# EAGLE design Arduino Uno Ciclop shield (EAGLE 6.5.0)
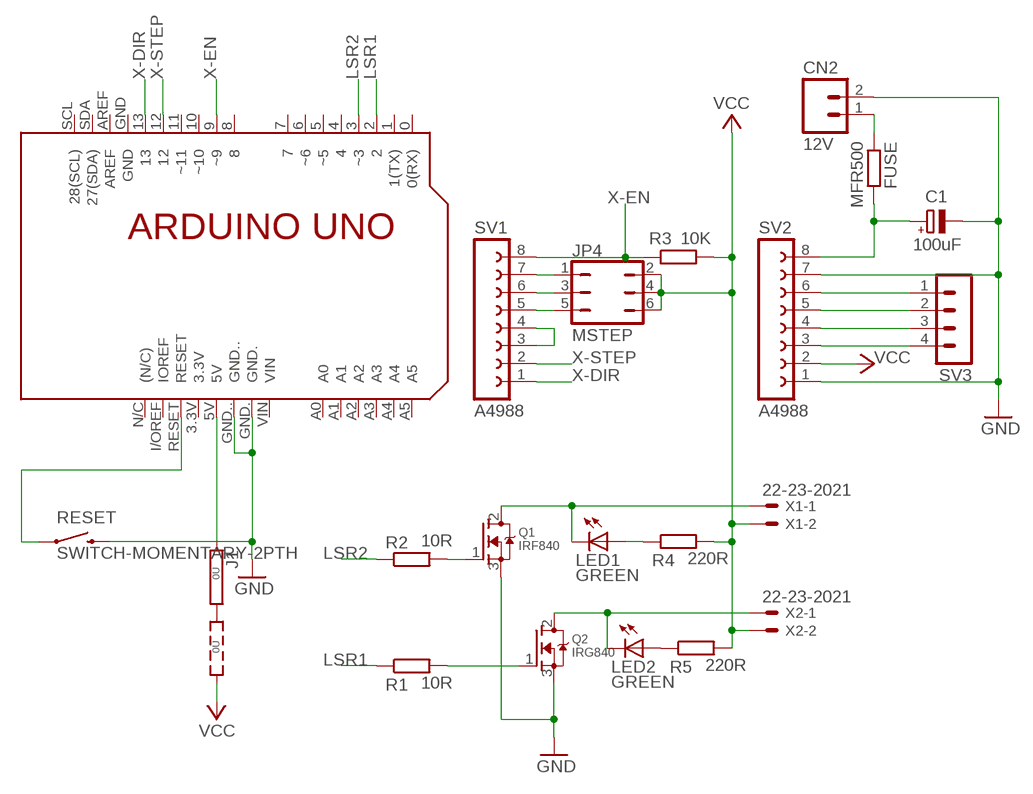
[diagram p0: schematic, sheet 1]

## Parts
C1  100uF  CPOL-EUB45181A  [B45181A]
CN2  12V  M025MM  [SCREWTERMINAL-5MM-2]
FUSE  MFR500  R-EU_0207/10  [0207/10]
J1  0R2  [0R2/10]
JP4  MSTEP  JP3Q  [JP3Q]
LED1  GREEN  LED5MM  [LED5MM]
LED2  GREEN  LED5MM  [LED5MM]
PCB1  ARDUINO_UNO  [ARDUINO_UNO]
Q1  IRF840  MOSFET-NGDS_TO220V  [TO220V]
Q2  IRG840  MOSFET-NGDS_TO220V  [TO220V]
R1  10R  R-EU_0207/10  [0207/10]
R2  10R  R-EU_0207/10  [0207/10]
R3  10K  R-EU_0207/10  [0207/10]
R4  220R  R-EU_0207/10  [0207/10]
R5  220R  R-EU_0207/10  [0207/10]
RESET  SWITCH-MOMENTARY-2PTH  [TACTILE-PTH]
SV1  A4988  FE08-1  [FE08]
SV2  A4988  FE08-1  [FE08]
SV3  MA04-1  [MA04-1]
X1  22-23-2021  [22-23-2021]
X2  22-23-2021  [22-23-2021]

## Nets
GND: C1.- CN2.2 PCB1.GND. PCB1.GND.. Q1.3(S) Q2.3(S) RESET.3 SV2.1 SV2.7
LSR1: PCB1.2 R1.1
LSR2: PCB1.3(~3) R2.1
N$1: LED2.A R5.1
N$2: SV2.6 SV3.1
N$3: SV2.5 SV3.2
N$4: SV2.4 SV3.3
N$5: SV2.3 SV3.4
N$6: Q1.1(G) R2.2
N$7: PCB1.RESET RESET.1
N$8: JP4.1 SV1.7
N$9: LED1.K(C) Q1.2(D) X1.1
N$10: JP4.3 SV1.6
N$11: JP4.5 SV1.5
N$12: C1.+ FUSE.2 SV2.8
N$13: CN2.1 FUSE.1
N$14: Q2.1(G) R1.2
N$15: SV1.3 SV1.4
N$16: LED2.K(C) Q2.2(D) X2.1
N$17: LED1.A R4.1
N$18: J1.1 PCB1.5V
VCC: J1.3 JP4.2 JP4.4 JP4.6 R3.2 R4.2 R5.2 SV2.2 X1.2 X2.2
X-DIR: PCB1.13 SV1.1
X-EN: PCB1.9(~9) R3.1 SV1.8
X-STEP: PCB1.12 SV1.2
Unconnected: J1.2 PCB1.0(0(RX)) PCB1.1(1(TX)) PCB1.3.3V PCB1.4 PCB1.5(~5) PCB1.6(~6) PCB1.7 PCB1.8 PCB1.10(~10) PCB1.11(~11) PCB1.A0 PCB1.A1 PCB1.A2 PCB1.A3 PCB1.A4 PCB1.A5 PCB1.AREF PCB1.GND PCB1.I/OREF(IOREF) PCB1.N/C((N/C)) PCB1.SCL(28(SCL)) PCB1.SDA(27(SDA)) PCB1.VIN

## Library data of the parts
C1 = rcl:CPOL-EU: POLARIZED CAPACITOR, European symbol
CN2 = SparkFun-Connectors:M02: Standard 2-pin 0.1" header. Use with; STOREFRONT_ID: PRT-08432
FUSE R1-R5 = resistor:R-EU_: RESISTOR, European symbol
J1 = jumper:0R2: Bridge switch 0R 2 x 10mm
JP4 = jumper:JP3Q: JUMPER
LED1 LED2 = led:LED: LED
PCB1 = E14_Arduino_revB:ARDUINO_UNO: Device for representing an Arduino Uno board with a footprint in an EAGLE design. Created by Dave Young for Element14. More EAGLE documentation at: http://www.element14.com/community/community/knode/cadsoft_eagle
Q1 Q2 = adafruit:MOSFET-N: N-Channel Mosfet 2N7002E - 60V 260mA SOT23 [Digikey: 2N7002ET1GOSTR-ND] - REEL BSH103 - 30V 850mA SOT23 [Digikey: 568-5013-1-ND]
RESET = SparkFun-Electromechanical:SWITCH-MOMENTARY-2: Various NO switches- pushbuttons, reed, etc; PROD_ID: SWCH-08441
SV1 SV2 = con-lsta:FE08-1: FEMALE HEADER; OC_FARNELL: unknown; OC_NEWARK: unknown
SV3 = con-lstb:MA04-1: PIN HEADER; OC_FARNELL: unknown; OC_NEWARK: unknown
X1 X2 = con-molex:22-23-2021: .100" (2.54mm) Center Header - 2 Pin; MF: MOLEX; MPN: 22-23-2021; OC_FARNELL: 1462926; OC_NEWARK: 25C3832

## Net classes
0 default: width 0.024 mm

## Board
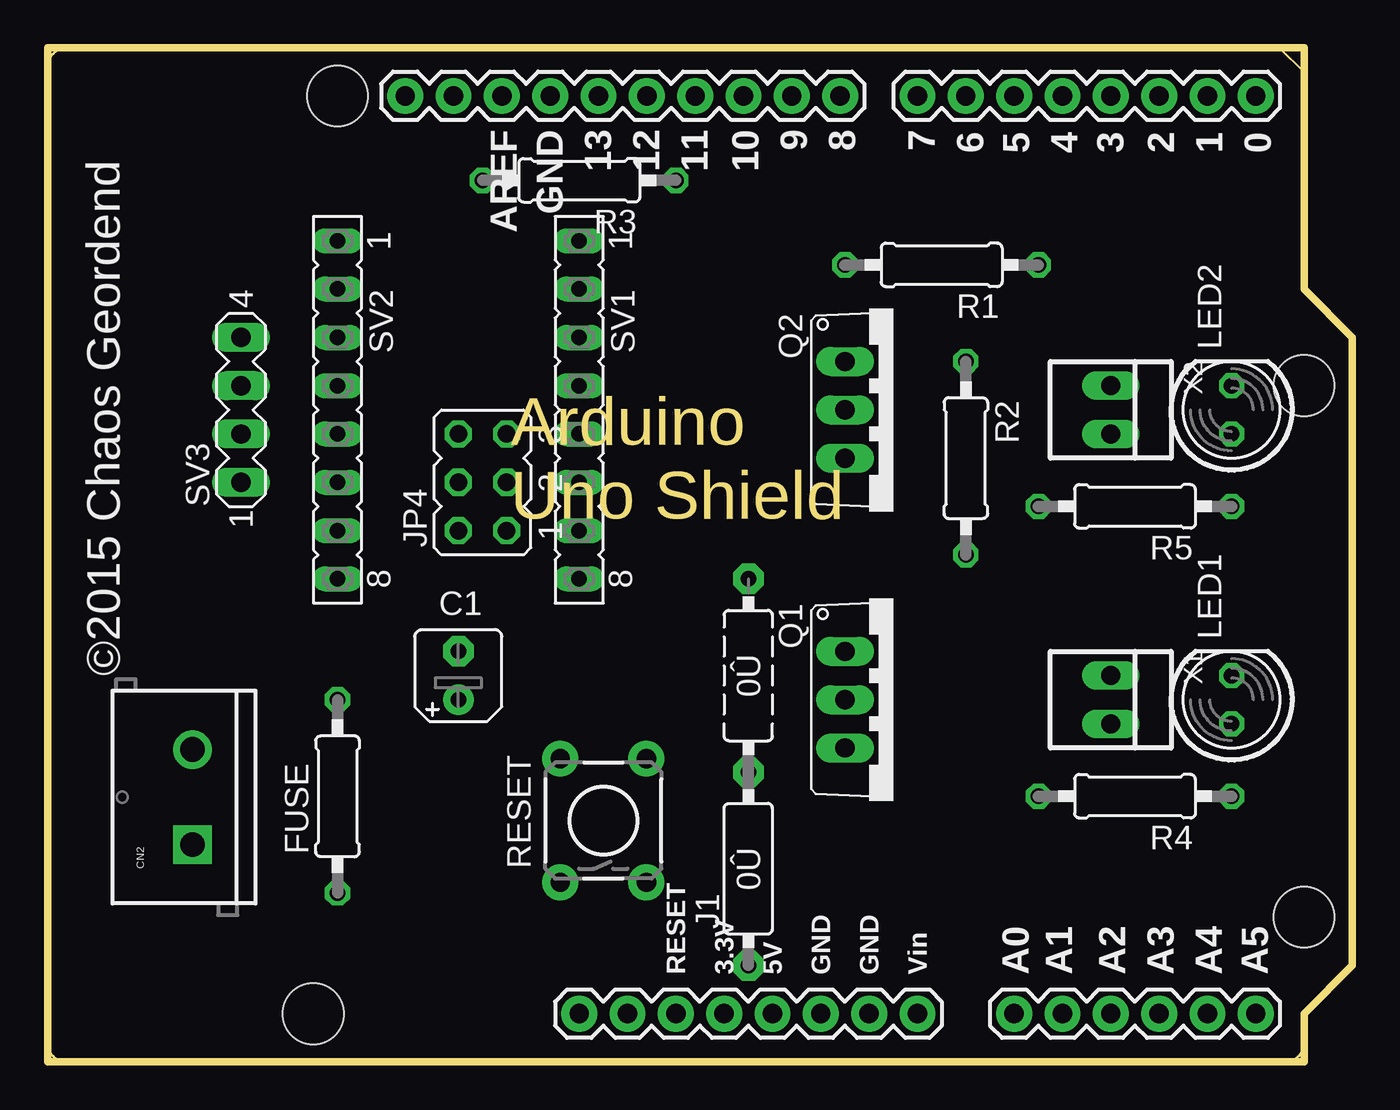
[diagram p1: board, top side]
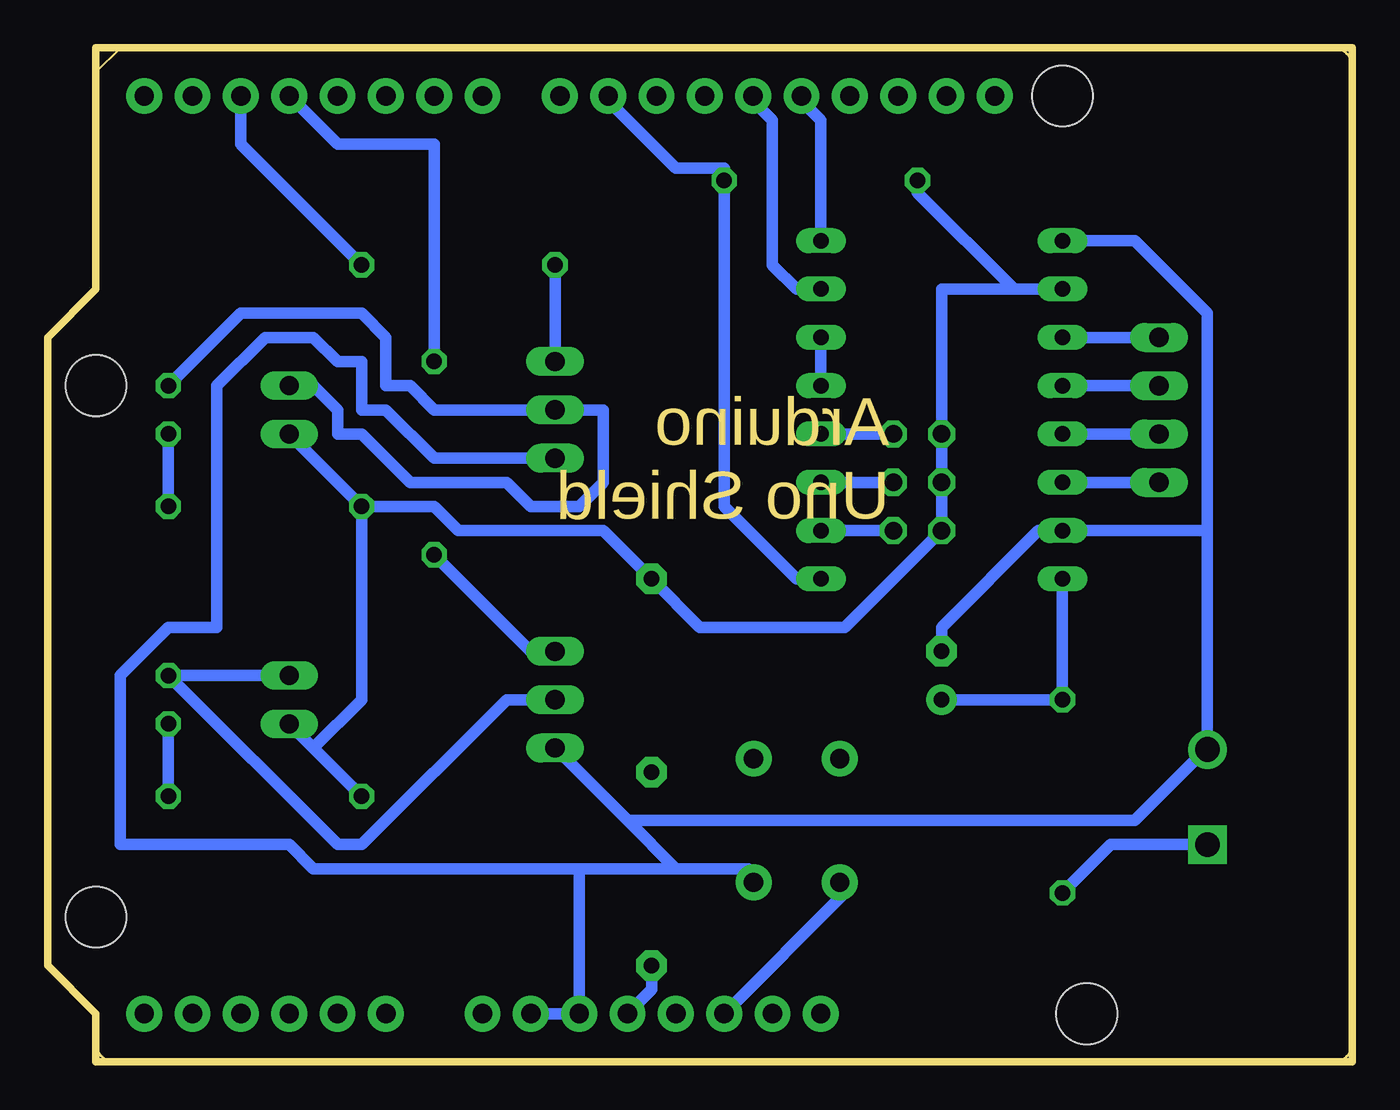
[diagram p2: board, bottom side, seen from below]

Size 68.58 x 53.34 mm. Coordinates in mm from the lower left corner, seen from the top.
Outline: 0,0 0,53.34 66.04,53.34 66.04,40.64 68.58,38.1 68.58,5.08 66.04,2.54 66.04,0 0,0
Copper layers (1*16): Top 0.035mm / dielectric 1.5mm / Bottom 0.035mm
Design rules "default *": minimum track width 24mil, minimum drill 24mil, track to track 16mil, track to pad 16mil, pad to pad 8mil, via to via 8mil, smd to smd 8mil, copper to edge 40mil, drill to drill 8mil, minimum pad ring 10mil, minimum via ring 8mil, stop-mask expansion 4mil, vias tented up to drill 0mil, thermal gap 10mil

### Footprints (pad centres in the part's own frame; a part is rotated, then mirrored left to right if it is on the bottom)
B45181A = drill 0.813 pad 1.6: + -1.27,0 | drill 0.813 pad 1.6 octagon: - 1.27,0
SCREWTERMINAL-5MM-2 = drill 1.3 pad 2.032 square: 1 0,0 | drill 1.3 pad 2.032: 2 5,0
0207/10 = drill 0.813 octagon: 1 -5.08,0; 2 5.08,0
0R2/10 = drill 0.813 pad 1.6 octagon: 1 -5.08,0; 2 5.08,0; 3 15.24,0
JP3Q = drill 0.914 octagon: 1 -2.54,-1.27; 2 -2.54,1.27; 3 0,-1.27; 4 0,1.27; 5 2.54,-1.27; 6 2.54,1.27
LED5MM = drill 0.813 octagon: A -1.27,0; K 1.27,0
ARDUINO_UNO = drill 1.016 pad 1.88: 0 63.5,50.8; 1 60.96,50.8; 2 58.42,50.8; 3 55.88,50.8; 3.3V 35.56,2.54; 4 53.34,50.8; 5 50.8,50.8; 5V 38.1,2.54; 6 48.26,50.8; 7 45.72,50.8; 8 41.656,50.8; 9 39.116,50.8; 10 36.576,50.8; 11 34.036,50.8; 12 31.496,50.8; 13 28.956,50.8; A0 50.8,2.54; A1 53.34,2.54; A2 55.88,2.54; A3 58.42,2.54; A4 60.96,2.54; A5 63.5,2.54; AREF 23.876,50.8; GND 26.416,50.8; GND. 43.18,2.54; GND.. 40.64,2.54; I/OREF 30.48,2.54; N/C 27.94,2.54; RESET 33.02,2.54; SCL 18.796,50.8; SDA 21.336,50.8; VIN 45.72,2.54 | hole 3.2: 66.04,7.62; 66.04,35.56; 15.24,50.8; 13.97,2.54
TO220V = drill 1.016 long: 1 -2.54,-2.54; 2 0,-2.54; 3 2.54,-2.54
TACTILE-PTH = drill 1.016 pad 1.88: 1 -3.251,2.261; 2 3.251,2.261; 3 -3.251,-2.261; 4 3.251,-2.261
FE08 = drill 0.813 long: 1 -8.89,0; 2 -6.35,0; 3 -3.81,0; 4 -1.27,0; 5 1.27,0; 6 3.81,0; 7 6.35,0; 8 8.89,0
MA04-1 = drill 1.016 long: 1 -3.81,0; 2 -1.27,0; 3 1.27,0; 4 3.81,0
22-23-2021 = drill 1 long: 1 -1.27,0; 2 1.27,0

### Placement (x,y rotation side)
C1  21.59,20.32 90 top
CN2  7.62,11.43 90 top
FUSE  15.24,13.97 90 top
J1  36.83,10.16 90 top
JP4  22.86,30.48 90 top
LED1  62.23,19.05 90 top
LED2  62.23,34.29 90 top
PCB1  0,0 0 top
Q1  44.45,19.05 270 top
Q2  44.45,34.29 270 top
R1  46.99,41.91 180 top
R2  48.26,31.75 270 top
R3  27.94,46.35 180 top
R4  57.15,13.97 180 top
R5  57.15,29.21 180 top
RESET  29.21,12.7 90 top
SV1  27.94,34.29 270 top
SV2  15.24,34.29 270 top
SV3  10.16,34.29 90 top
X1  55.88,19.05 270 top
X2  55.88,34.29 270 top

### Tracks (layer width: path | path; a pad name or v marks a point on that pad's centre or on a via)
GND
  Bottom 0.61: C1.- 21.59,22.86 16.51,27.94 SV2.7 7.62,27.94 | SV2.1 11.43,43.18 7.62,39.37 7.62,27.94 | 7.62,27.94 7.62,16.51 | PCB1.GND. PCB1.GND.. 40.64,10.16 | 35.56,10.16 38.1,12.7 | 38.1,12.7 Q1.3 | 35.56,10.16 31.75,10.16 RESET.3 | Q2.3 48.26,31.75 50.8,34.29 52.07,34.29 52.07,36.83 53.34,36.83 54.61,38.1 57.15,38.1 59.69,35.56 59.69,22.86 62.23,22.86 64.77,20.32 64.77,11.43 55.88,11.43 54.61,10.16 40.64,10.16 | 35.56,10.16 40.64,10.16 | 7.62,16.51 11.43,12.7 38.1,12.7 | 7.62,16.51 CN2.2
LSR1
  Bottom 0.61: R1.1 58.42,48.26 PCB1.2
LSR2
  Bottom 0.61: R2.1 48.26,48.26 53.34,48.26 PCB1.3
N$1
  Bottom 0.61: LED2.A R5.1
N$2
  Bottom 0.61: SV3.1 SV2.6
N$3
  Bottom 0.61: SV3.2 SV2.5
N$4
  Bottom 0.61: SV3.3 SV2.4
N$5
  Bottom 0.61: SV3.4 SV2.3
N$6
  Bottom 0.61: R2.2 43.18,21.59 Q1.1
N$7
  Bottom 0.61: PCB1.RESET 26.67,8.89 RESET.1
N$8
  Bottom 0.61: JP4.1 SV1.7
N$9
  Bottom 0.61: X1.1 LED1.K 53.34,11.43 52.07,11.43 44.45,19.05 Q1.2
N$10
  Bottom 0.61: JP4.3 SV1.6
N$11
  Bottom 0.61: JP4.5 SV1.5
N$12
  Bottom 0.61: SV2.8 FUSE.2 C1.+
N$13
  Bottom 0.61: FUSE.1 12.7,11.43 CN2.1
N$14
  Bottom 0.61: Q2.1 R1.2
N$15
  Bottom 0.61: SV1.3 SV1.4
N$16
  Bottom 0.61: LED2.K 58.42,39.37 52.07,39.37 50.8,38.1 50.8,35.56 49.53,35.56 48.26,34.29 Q2.2 39.37,34.29 39.37,30.48 40.64,29.21 43.18,29.21 44.45,30.48 49.53,30.48 52.07,33.02 53.34,33.02 53.34,34.29 54.61,35.56 X2.1
N$17
  Bottom 0.61: LED1.A R4.1
N$18
  Bottom 0.61: J1.1 36.83,3.81 PCB1.5V
VCC
  Bottom 0.61: 17.78,40.64 SV2.2 | 17.78,40.64 22.86,45.72 R3.2 | 17.78,40.64 21.59,40.64 JP4.6 JP4.4 JP4.2 26.67,22.86 34.29,22.86 J1.3 39.37,27.94 46.99,27.94 48.26,29.21 R5.2 | X1.2 54.61,16.51 | 54.61,16.51 R4.2 | X2.2 R5.2 | 54.61,16.51 52.07,19.05 R5.2
X-DIR
  Bottom 0.61: SV1.1 27.94,49.53 29.21,50.8 PCB1.13
X-EN
  Bottom 0.61: SV1.8 29.21,25.4 33.02,29.21 R3.1 33.02,46.99 35.56,46.99 39.37,50.8 PCB1.9
X-STEP
  Bottom 0.61: SV1.2 29.21,40.64 30.48,41.91 30.48,49.53 31.75,50.8 PCB1.12

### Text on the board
tPlace: ©2015 Chaos Geordend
